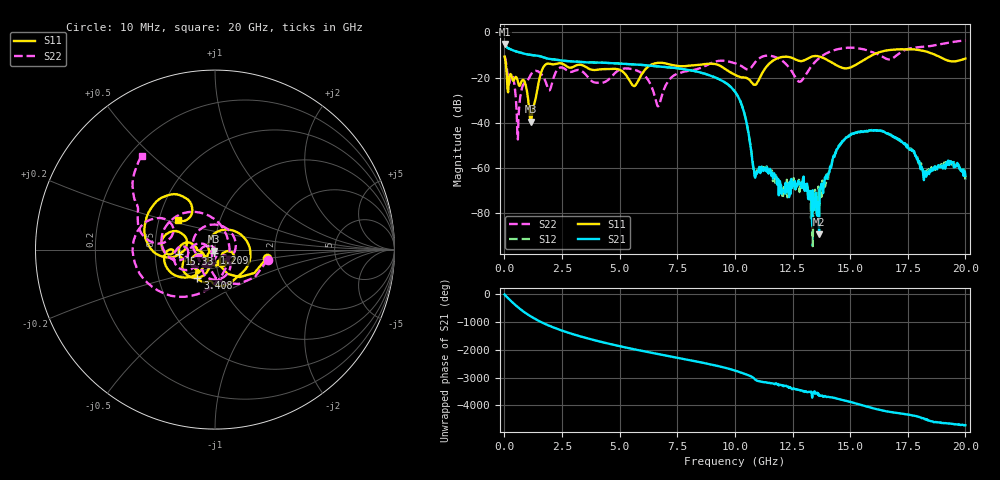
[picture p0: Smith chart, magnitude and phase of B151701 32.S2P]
!  2-Port S-parameters saved by WinCal
! VAR MeasName=S-Parameters (CALIBRATED_DATA) read from VNA (N5244A)
! VAR MeasDate=2015-12-24 19:13:00
! VAR NAME=B151701 32
! VAR FILENAME=B151701 32.S2P
! VAR DATE=2015-12-24 19:13:00
! VAR PHYS_PORTS=1,3
# Hz S DB R 50
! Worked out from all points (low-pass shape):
!   801 points, 10 MHz to 20 GHz, reference 50 ohm
!   highest |S21| = -5.13 dB at 10 MHz (marker M1); lowest = -89.5 dB at 13.65 GHz (marker M2)
!   |S21| within 3 dB of the highest: start of sweep to 413.4 MHz
!   lowest |S11| = -39.6 dB at 1.134 GHz (marker M3), VSWR 1.02, Z = 49.3 - j0.777 ohm
!   |S11| at or under -10 dB: start of sweep to 15.98 GHz; 18.7 GHz to end of sweep
!   |S22| runs from -47.4 to -3.6 dB; largest |S21 - S12| = 0.0022
!   S11 on the Smith chart (normalised r, x): 10 MHz: 1.80, -0.19; 1.209 GHz: 0.99, -0.03; 3.408 GHz: 0.78, -0.26; 15.33 GHz: 0.66, -0.04; 20 GHz: 0.63, +0.22
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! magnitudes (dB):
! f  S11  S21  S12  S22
! 10 MHz  -10.7  -5.1  -5.2  -10.5
! 584.7 MHz  -21.8  -8.7  -8.7  -47.4
! 884.6 MHz  -22.0  -9.5  -9.5  -22.4
! 1.134 GHz  -39.6  -10.0  -10.0  -18.9
! 1.209 GHz  -35.6  -10.1  -10.1  -17.8
! 1.759 GHz  -14.5  -11.3  -11.3  -21.1
! 3.358 GHz  -14.4  -13.2  -13.2  -17.1
! 3.408 GHz  -14.6  -13.2  -13.2  -17.5
! 5.782 GHz  -21.9  -14.3  -14.3  -17.1
! 6.682 GHz  -13.5  -15.1  -15.1  -32.7
! 7.431 GHz  -14.7  -15.8  -15.8  -18.6
! 10.01 GHz  -18.8  -26.3  -26.3  -13.7
! 10.43 GHz  -20.0  -36.7  -36.6  -15.9
! 10.9 GHz  -23.2  -63.3  -61.7  -12.9
! 12.8 GHz  -12.6  -66.4  -70.7  -21.8
! 13.35 GHz  -10.7  -85.5  -74.6  -14.5
! 13.65 GHz  -10.6  -89.5  -76.0  -11.5
! 14.5 GHz  -15.1  -50.3  -50.2  -7.3
! 15.33 GHz  -13.9  -44.1  -44.0  -7.0
! 16.68 GHz  -7.8  -44.9  -44.9  -12.0
! 18.25 GHz  -8.4  -61.4  -61.8  -6.3
! 20 GHz  -11.6  -63.5  -65.2  -3.6
